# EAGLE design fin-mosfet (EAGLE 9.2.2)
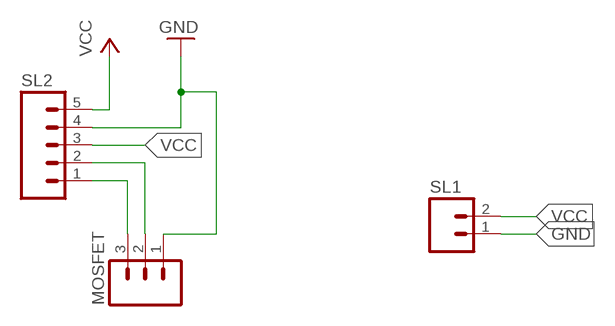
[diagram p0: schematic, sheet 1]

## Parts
MOSFET  M03  [03P]
SL1  M02  [02P]
SL2  M05  [05P]

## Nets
GND: MOSFET.1 SL1.1 SL2.4
N$1: MOSFET.3 SL2.1
N$3: MOSFET.2 SL2.2
VCC: SL1.2 SL2.3 SL2.5

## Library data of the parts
MOSFET = con-amp-quick:M03: AMP QUICK CONNECTOR; OC_FARNELL: unknown; OC_NEWARK: unknown
SL1 = con-amp-quick:M02: AMP QUICK CONNECTOR; OC_FARNELL: unknown; OC_NEWARK: unknown
SL2 = con-amp-quick:M05: AMP QUICK CONNECTOR; OC_FARNELL: unknown; OC_NEWARK: unknown

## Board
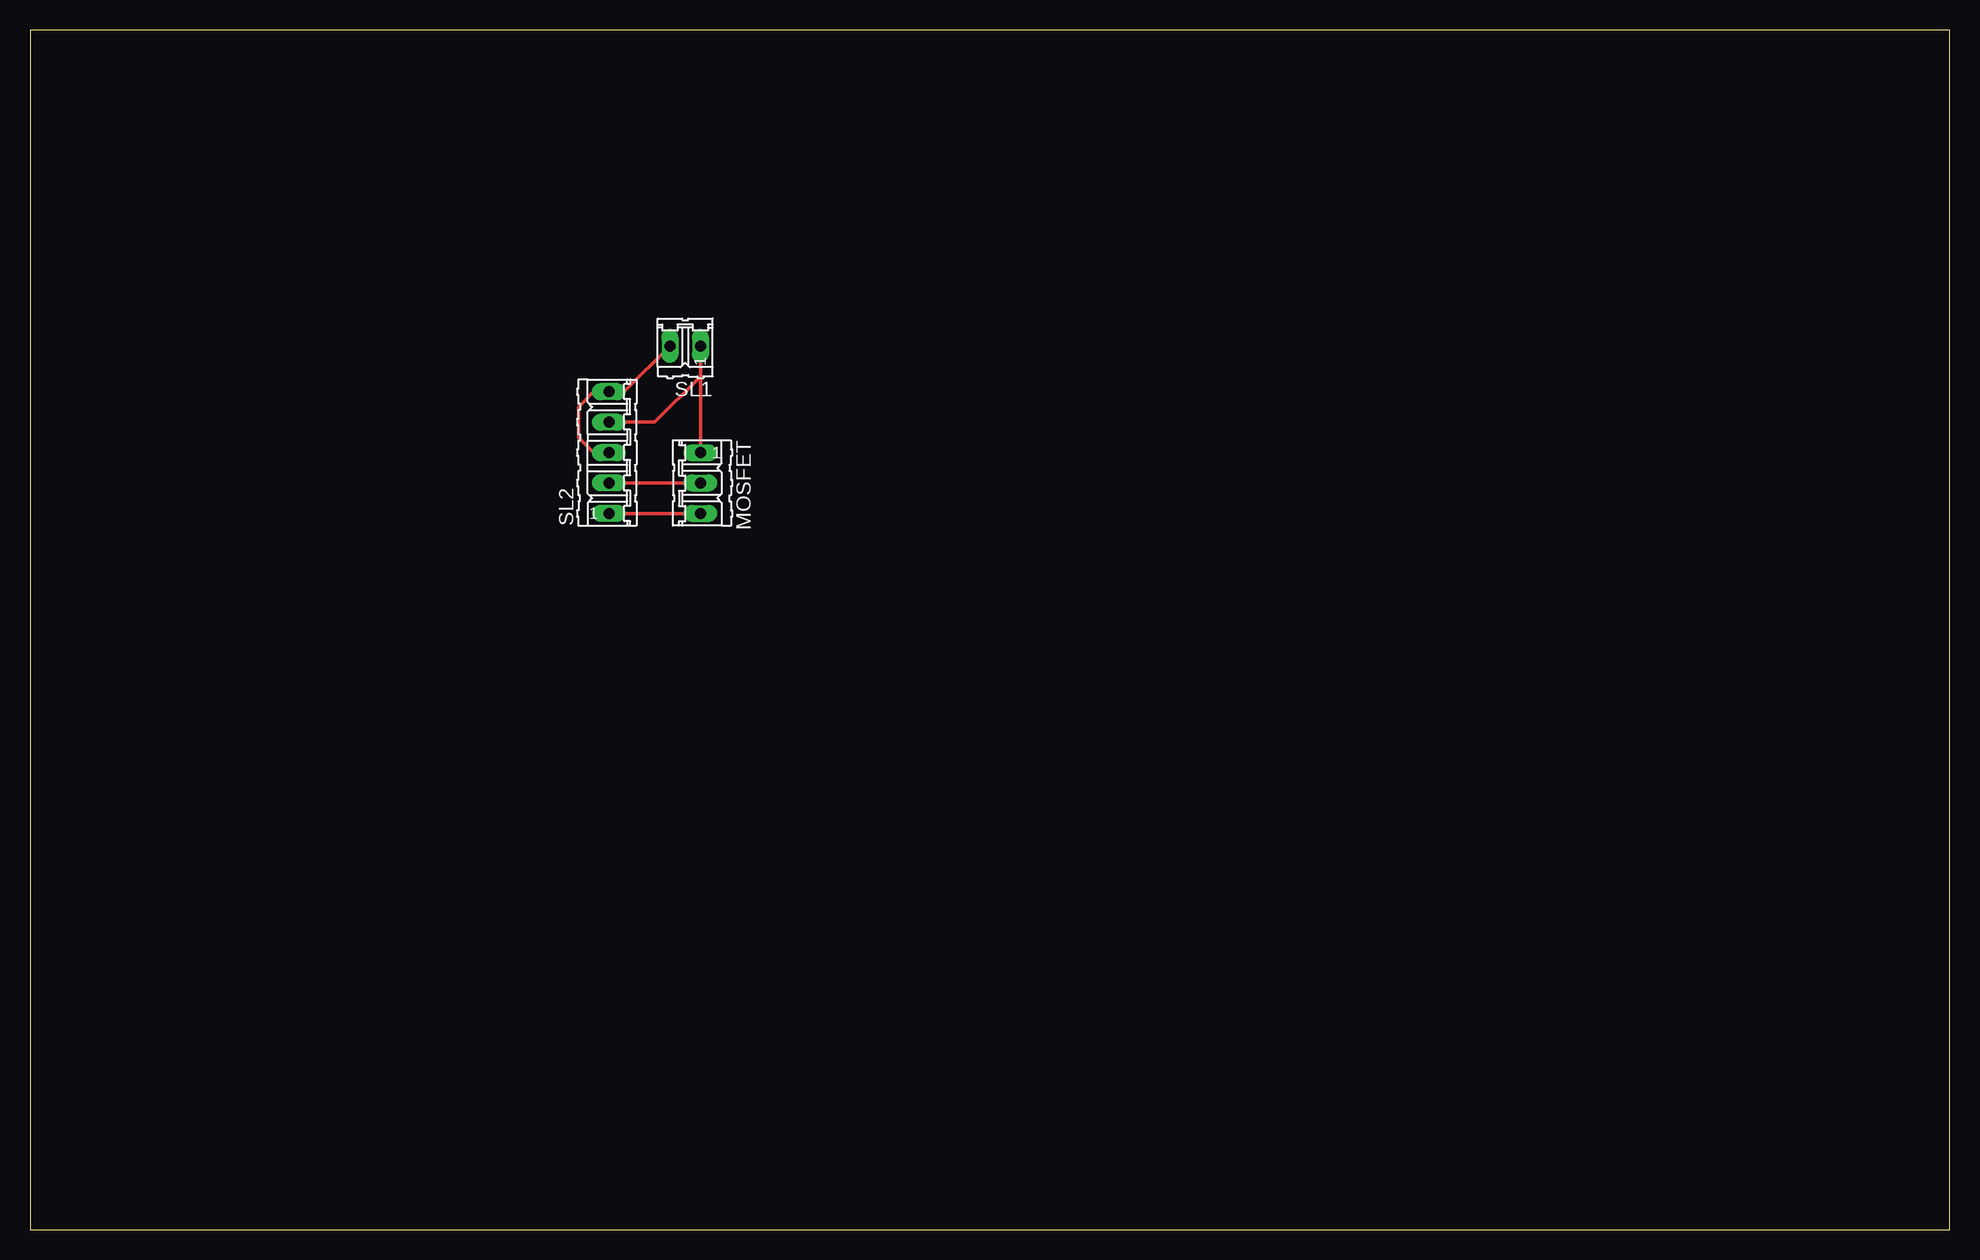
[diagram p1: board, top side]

Size 160 x 100 mm. Coordinates in mm from the lower left corner, seen from the top.
Outline: 0,0 160,0 160,100 0,100 0,0
Copper layers (1*16): Top 0.035mm / dielectric 1.5mm / Bottom 0.035mm
Design rules "default": minimum track width 6mil, minimum drill 0.35mm, track to track 6mil, track to pad 6mil, pad to pad 6mil, via to via 6mil, smd to smd 6mil, copper to edge 40mil, drill to drill 6mil, minimum pad ring 10mil, minimum via ring 8mil, stop-mask expansion 4mil, vias tented up to drill 0mil, thermal gap 10mil

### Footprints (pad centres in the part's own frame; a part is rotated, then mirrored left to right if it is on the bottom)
03P = drill 0.914 long: 1 -2.54,0; 2 0,0; 3 2.54,0
02P = drill 0.914 long: 1 -1.27,0; 2 1.27,0
05P = drill 0.914 long: 1 -5.08,0; 2 -2.54,0; 3 0,0; 4 2.54,0; 5 5.08,0

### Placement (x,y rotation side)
MOSFET  55.88,62.23 270 top
SL1  54.61,73.66 180 top
SL2  48.26,64.77 90 top

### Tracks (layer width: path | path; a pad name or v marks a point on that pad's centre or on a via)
GND
  Top 0.305: SL2.4 52.07,67.31 55.88,71.12 | 55.88,71.12 SL1.1 | MOSFET.1 55.88,71.12
N$1
  Top 0.305: MOSFET.3 SL2.1
N$3
  Top 0.305: SL2.2 MOSFET.2
VCC
  Top 0.305: SL1.2 49.53,69.85 SL2.5 46.99,69.85 45.72,68.58 45.72,66.04 46.99,64.77 SL2.3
